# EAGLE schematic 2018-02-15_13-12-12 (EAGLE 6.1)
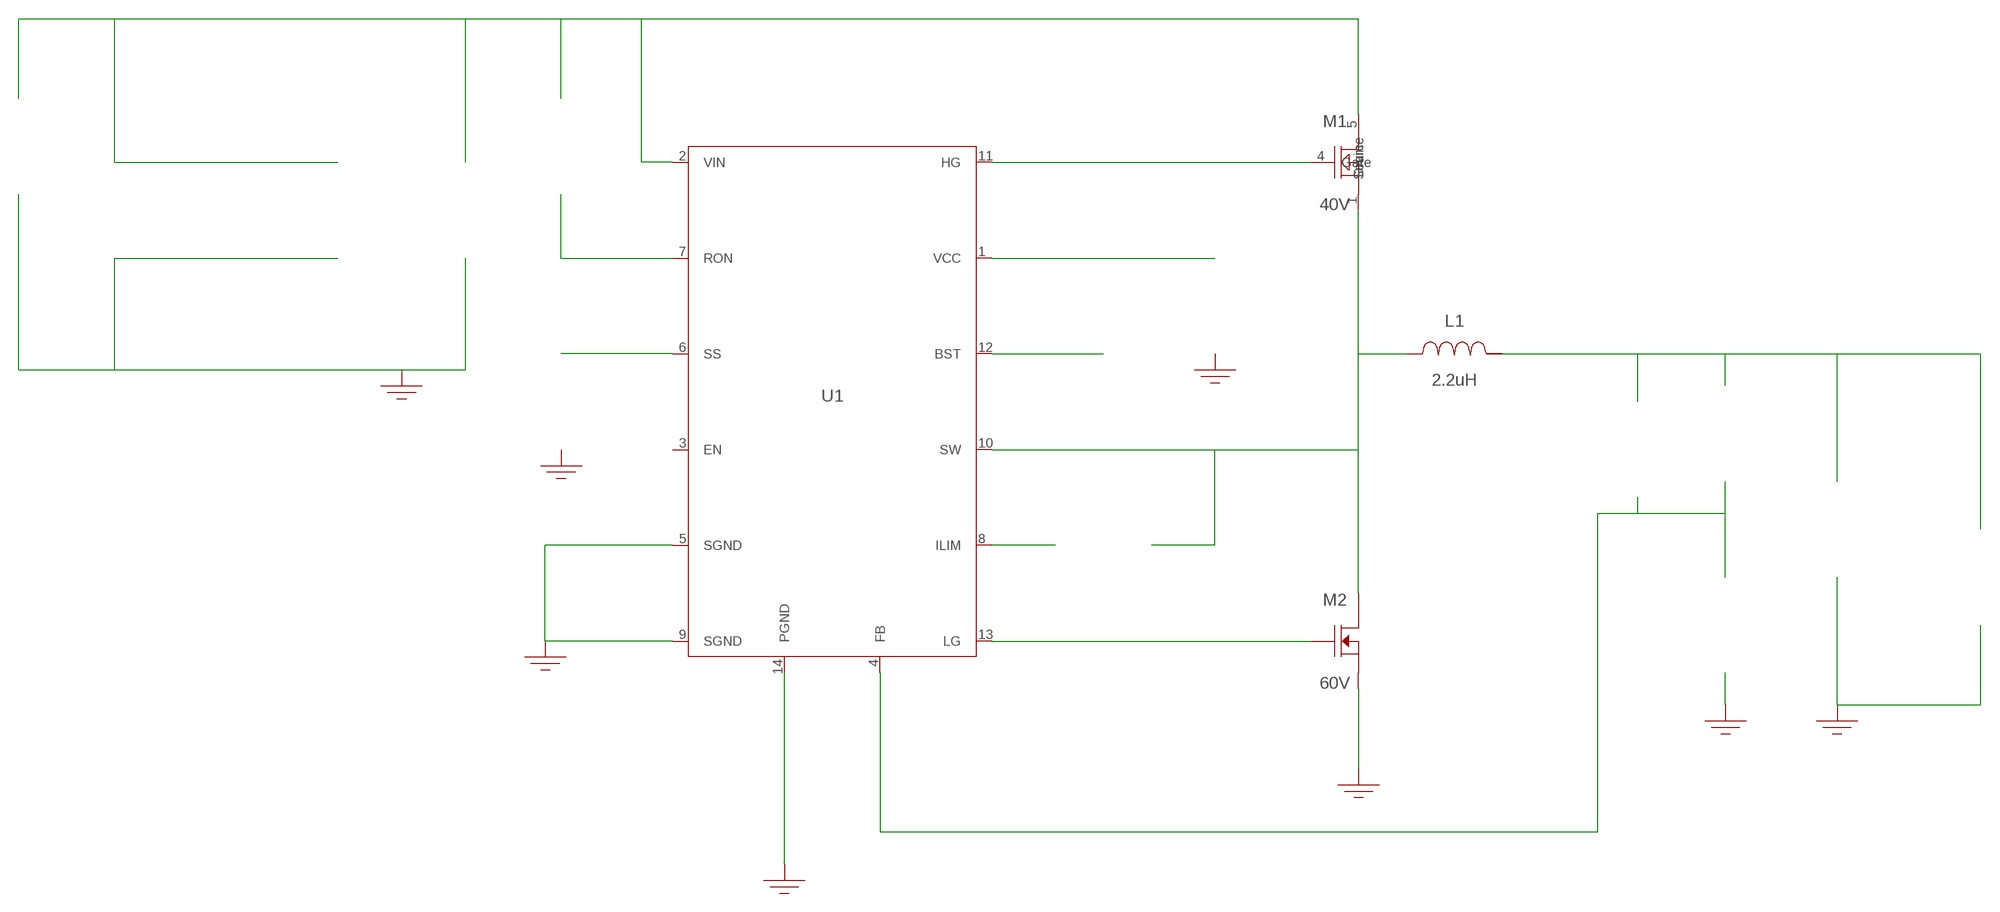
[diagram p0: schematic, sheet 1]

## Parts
CBST  680nF  ECPU1C684MA5ECPU1C684MA5  [1206]  (not placed on a sheet)
CBYP  100nF  08055C104MAT2A08055C104MAT2A  [0805]  (not placed on a sheet)
CFF  470pF  C0805C471K5RACTUC0805C471K5RACTU  [0805]  (not placed on a sheet)
CIN  22uF  C2012X5R1V226M125ACC2012X5R1V226M125AC  [0805]  (not placed on a sheet)
CIN_2  22uF  C2012X5R1V226M125ACC2012X5R1V226M125AC  [0805]  (not placed on a sheet)
CIN_3  22uF  C2012X5R1V226M125ACC2012X5R1V226M125AC  [0805]  (not placed on a sheet)
COUT  220uF  6SVPE220MW6SVPE220MW  [CAPSMT_62_E61]  (not placed on a sheet)
CSS  15nF  C2012C0G1H153J085AAC2012C0G1H153J085AA  [0805]  (not placed on a sheet)
CVCC  1uF  ECPU1C105MA5ECPU1C105MA5  [1210]  (not placed on a sheet)
GND1  WB_GND  WB_GNDWB_GND  [WB_GND]
GND2  WB_GND  WB_GNDWB_GND  [WB_GND]
GND3  WB_GND  WB_GNDWB_GND  [WB_GND]
GND4  WB_GND  WB_GNDWB_GND  [WB_GND]
GND5  WB_GND  WB_GNDWB_GND  [WB_GND]
GND6  WB_GND  WB_GNDWB_GND  [WB_GND]
GND7  WB_GND  WB_GNDWB_GND  [WB_GND]
GND8  WB_GND  WB_GNDWB_GND  [WB_GND]
IOUT  WB_CURRENT_LOAD  WB_CURRENT_LOADWB_CURRENT_LOAD  [WB_CURRENT_LOAD]  (not placed on a sheet)
L1  2.2uH  XAL1010-222MEBXAL1010-222MEB  [XAL1010]
M1  40V  CSD18504Q5ACSD18504Q5A  [TRANS_NexFET_Q5A]
M2  60V  CSD18531Q5ACSD18531Q5A  [TRANS_NexFET_Q5A]
RFB1  10k  RR1220P-103-DRR1220P-103-D  [0805]  (not placed on a sheet)
RFB2  73.2k  ERJ-6ENF7322VERJ-6ENF7322V  [0805]  (not placed on a sheet)
RILIM  2.05k  ERJ-6ENF2051VERJ-6ENF2051V  [0805]  (not placed on a sheet)
RON  107k  ERJ-6ENF1073VERJ-6ENF1073V  [0805]  (not placed on a sheet)
U1  LM3150MH/NOPB  LM3150MH/NOPBLM3150MH/NOPB  [MXA14A]
VIN  WB_BATTERY  WB_BATTERYWB_BATTERY  [WB_BATTERY]  (not placed on a sheet)

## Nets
0: Cbyp.2@2 Cin.2@2 Cin_2.2@2 Cin_3.2@2 Cout.-@2 Css.2@2 Cvcc.2@2 GND1.1 GND2.1 GND3.1 GND4.1 GND5.1 GND6.1 GND7.1 GND8.1 Iout.-@2 M2.1(Source) M2.2(Source) M2.3(Source) Rfb1.2@2 U1.5(SGND) U1.9(SGND) U1.14(PGND) U1.15(DAP) Vin.-@2
1: Css.1@1 U1.6(SS)
2: Cbyp.1@1 Cin.1@1 Cin_2.1@1 Cin_3.1@1 M1.5(Drain) M1.6(Drain) M1.7(Drain) M1.8(Drain) M1.9(Drain) Ron.1@1 U1.2(VIN) Vin.+@1
3: Ron.2@2 U1.7(RON)
4: Cff.1@1 Cout.+@1 Iout.+@1 L1.2 Rfb2.1@1
5: Cff.2@2 Rfb1.1@1 Rfb2.2@2 U1.4(FB)
6: Cbst.2@2 L1.1 M1.1(Source) M1.2(Source) M1.3(Source) M2.5(Drain) M2.6(Drain) M2.7(Drain) M2.8(Drain) M2.9(Drain) Rilim.1@1 U1.10(SW)
7: M2.4(Gate) U1.13(LG)
8: M1.4(Gate) U1.11(HG)
9: Cbst.1@1 U1.12(BST)
10: Cvcc.1@1 U1.1(VCC)
11: Rilim.2@2 U1.8(ILIM)
Unconnected: CBST.1 CBST.2 CBYP.1 CBYP.2 CFF.1 CFF.2 CIN.1 CIN.2 CIN_2.1 CIN_2.2 CIN_3.1 CIN_3.2 COUT.1(+) COUT.2(-) CSS.1 CSS.2 CVCC.1 CVCC.2 IOUT.1(+) IOUT.2(-) RFB1.1 RFB1.2 RFB2.1 RFB2.2 RILIM.1 RILIM.2 RON.1 RON.2 U1.3(EN) VIN.1(+) VIN.2(-)

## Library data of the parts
CBST = AcceleratedDesigns_Lib:ECPU1C684MA5; Cap: 6.8E-7; Datasheet_URL: http://www.panasonic.com/industrial/components/pdf/ef038%5Fecpu%5Fdne.pdf; ESR: 0.0; IRMS: 0.0; Manufacturer_Name: Panasonic; Manufacturer_Part_Number: ECPU1C684MA5; VDC: 16.0; Vendor: Panasonic
CBYP = AcceleratedDesigns_Lib:08055C104MAT2A; Cap: 1.0E-7; ESR: 0.024; IRMS: 0.0; Manufacturer_Name: AVX; Manufacturer_Part_Number: 08055C104MAT2A; VDC: 50.0; Vendor: AVX
CFF = AcceleratedDesigns_Lib:C0805C471K5RACTU; Cap: 4.7E-10; ESR: 0.688; IRMS: 0.213; Manufacturer_Name: Kemet; Manufacturer_Part_Number: C0805C471K5RACTU; VDC: 50.0; Vendor: Kemet
CIN CIN_2 CIN_3 = AcceleratedDesigns_Lib:C2012X5R1V226M125AC; Cap: 2.2E-5; Datasheet_URL: https://product.tdk.com/en/search/capacitor/ceramic/mlcc/info?part%5Fno%3DC2012X5R1V226M125AC; ESR: 0.00205; IRMS: 4.55587; Manufacturer_Name: TDK; Manufacturer_Part_Number: C2012X5R1V226M125AC; VDC: 35.0; Vendor: TDK
COUT = AcceleratedDesigns_Lib:6SVPE220MW; Cap: 2.2E-4; Datasheet_URL: http://industrial.panasonic.com/www%2Ddata/pdf/AAB8000/AAB8000CE2.pdf; ESR: 0.015; IRMS: 3.15; Manufacturer_Name: Panasonic; Manufacturer_Part_Number: 6SVPE220MW; VDC: 6.3; Vendor: Panasonic
CSS = AcceleratedDesigns_Lib:C2012C0G1H153J085AA; Cap: 1.5E-8; Datasheet_URL: http://product.tdk.com/capacitor/mlcc/en/documents/mlcc%5Fcommercial%5Fgeneral%5Fen.pdf; ESR: 0.0; IRMS: 0.0; Manufacturer_Name: TDK; Manufacturer_Part_Number: C2012C0G1H153J085AA; VDC: 50.0; Vendor: TDK
CVCC = AcceleratedDesigns_Lib:ECPU1C105MA5; Cap: 1.0E-6; Datasheet_URL: http://www.panasonic.com/industrial/components/pdf/ef038%5Fecpu%5Fdne.pdf; ESR: 0.0; IRMS: 0.0; Manufacturer_Name: Panasonic; Manufacturer_Part_Number: ECPU1C105MA5; VDC: 16.0; Vendor: Panasonic
GND1-GND8 = AcceleratedDesigns_Lib:WB_GND; Manufacturer_Name: WB_GND; Manufacturer_Part_Number: WB_GND; PowerPortType: POWER_GROUND; Value: Value
IOUT = AcceleratedDesigns_Lib:WB_CURRENT_LOAD; Manufacturer_Name: WB_CURRENT_LOAD; Manufacturer_Part_Number: WB_CURRENT_LOAD; PowerPortType: POWER_GROUND; Value: Value
L1 = AcceleratedDesigns_Lib:XAL1010-222MEB; DCR: 0.00255; Datasheet_URL: http://www.coilcraft.com/pdfs/xal1010.pdf; IDC: 32.0; L: 2.2E-6; Manufacturer_Name: Coilcraft; Manufacturer_Part_Number: XAL1010-222MEB; Vendor: Coilcraft
M1 = AcceleratedDesigns_Lib:CSD18504Q5A; Datasheet_URL: http://www.ti.com/lit/ds/symlink/csd18504q5a.pdf; IdsMax: 50.0; Manufacturer_Name: Texas Instruments; Manufacturer_Part_Number: CSD18504Q5A; QgTyp: 7.7; Quantity: 1; Rdson45: 0.0098; VdsMax: 40.0; Vendor: Texas Instruments
M2 = AcceleratedDesigns_Lib:CSD18531Q5A; Datasheet_URL: http://www.ti.com/lit/ds/symlink/csd18531q5a.pdf; IdsMax: 100.0; Manufacturer_Name: Texas Instruments; Manufacturer_Part_Number: CSD18531Q5A; QgTyp: 18.0; Quantity: 1; Rdson45: 0.0058; VdsMax: 60.0; Vendor: Texas Instruments
RFB1 = AcceleratedDesigns_Lib:RR1220P-103-D; Manufacturer_Name: Susumu Co Ltd; Manufacturer_Part_Number: RR1220P-103-D; Power: 0.1; Resistance: 10000.0; Tolerance: 0.5; Vendor: Susumu Co Ltd
RFB2 = AcceleratedDesigns_Lib:ERJ-6ENF7322V; Manufacturer_Name: Panasonic; Manufacturer_Part_Number: ERJ-6ENF7322V; Power: 0.125; Resistance: 73200.0; Tolerance: 1.0; Vendor: Panasonic
RILIM = AcceleratedDesigns_Lib:ERJ-6ENF2051V; Manufacturer_Name: Panasonic; Manufacturer_Part_Number: ERJ-6ENF2051V; Power: 0.125; Resistance: 2050.0; Tolerance: 1.0; Vendor: Panasonic
RON = AcceleratedDesigns_Lib:ERJ-6ENF1073V; Manufacturer_Name: Panasonic; Manufacturer_Part_Number: ERJ-6ENF1073V; Power: 0.125; Resistance: 107000.0; Tolerance: 1.0; Vendor: Panasonic
U1 = AcceleratedDesigns_Lib:LM3150MH/NOPB; Datasheet_URL: http://www.ti.com/product/lm3150; Frequency: 1000000.0; Imax: 12.0; Manufacturer_Name: Texas Instruments; Manufacturer_Part_Number: LM3150MH/NOPB; Mktg_Package: NA; NSID: LM3150MH/NOPB; Package: NA; Vendor: Texas Instruments
VIN = AcceleratedDesigns_Lib:WB_BATTERY; Manufacturer_Name: WB_BATTERY; Manufacturer_Part_Number: WB_BATTERY; PowerPortType: POWER_GROUND; Value: Value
